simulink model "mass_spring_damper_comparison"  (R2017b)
settings: Solver=FixedStepAuto  StartTime=0.0  StopTime=10.0  FixedStep=time  RelTol=1e-3
undefined symbols (not defined in the file): m

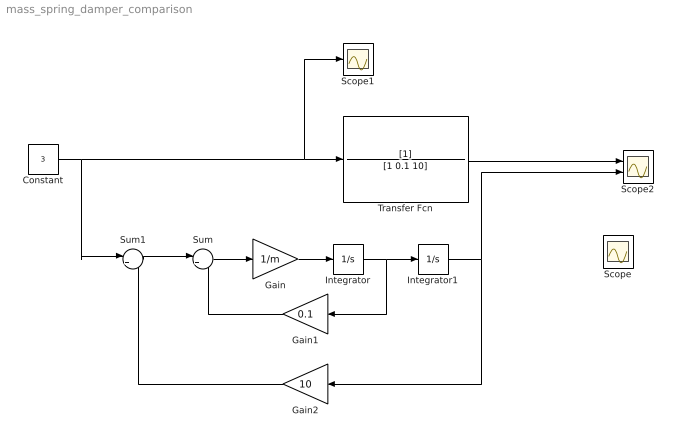
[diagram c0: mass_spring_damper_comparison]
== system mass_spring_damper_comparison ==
  Constant : Constant  Value=3
  Gain : Gain  Gain=1/m
  Gain1 : Gain  Gain=0.1
  Gain2 : Gain  Gain=10
  Integrator : Integrator
  Integrator1 : Integrator
  Scope : Scope  NumInputPorts=2
  Scope1 : Scope
  Scope2 : Scope  NumInputPorts=2
  Sum : Sum  Inputs=|+-
  Sum1 : Sum  Inputs=|+-
  Transfer Fcn : TransferFcn  Denominator=[1 0.1 10]
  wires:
  Transfer Fcn/1 -> Scope2/1
  Gain1/1 -> Sum/2
  Integrator1/1 -> Scope2/2, Gain2/1
  Sum1/1 -> Sum/1
  Integrator/1 -> Gain1/1, Integrator1/1
  Gain2/1 -> Sum1/2
  Sum/1 -> Gain/1
  Constant/1 -> Sum1/1, Scope1/1, Transfer Fcn/1
  Gain/1 -> Integrator/1
